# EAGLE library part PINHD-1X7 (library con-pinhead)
PIN HEADER
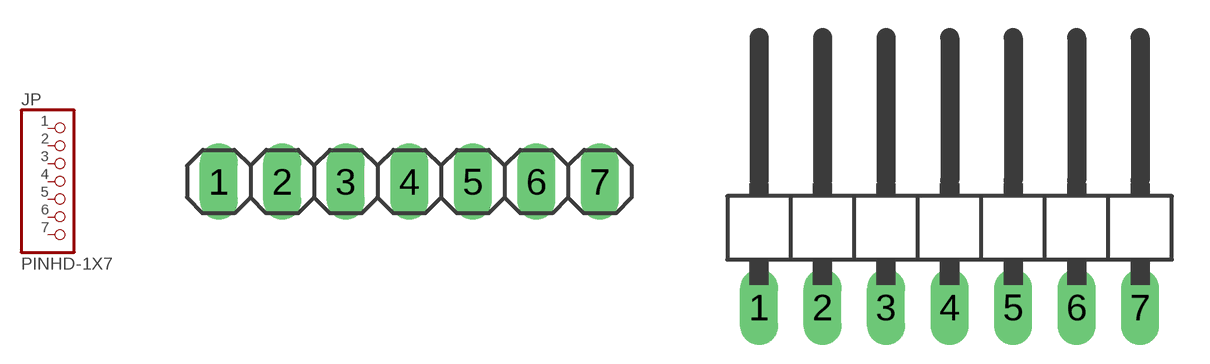
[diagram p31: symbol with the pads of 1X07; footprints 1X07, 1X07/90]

Designator prefix JP

## PINHD-1X7_2.54  [1X07]
1  1  pas
2  2  pas
3  3  pas
4  4  pas
5  5  pas
6  6  pas
7  7  pas

## PINHD-1X7_2.54-90°  [1X07/90]
Pads as for 1X07

## PINHD-1X7_2.00  [1X07M]
Pads as for 1X07

## PINHD-1X7_2.54-SMD  [1X07SMD]
Pads as for 1X07

## PINHD-1X7_2.54-SMD-90°  [1X07SMD/90]
Pads as for 1X07

## Footprint 1X07 (pad centres in mm)
PIN HEADER - 2.54
drill 1.016 long: 1 -7.62,0; 2 -5.08,0; 3 -2.54,0; 4 0,0; 5 2.54,0; 6 5.08,0; 7 7.62,0

## Footprint 1X07/90 (pad centres in mm)
PIN HEADER - 2.54 90°
drill 1.016 long: 1 -7.62,-3.81; 2 -5.08,-3.81; 3 -2.54,-3.81; 4 0,-3.81; 5 2.54,-3.81; 6 5.08,-3.81; 7 7.62,-3.81

## Footprint 1X07M (pad centres in mm)
PIN HEADER - 2
drill 0.914 square: 1 -6,0
drill 0.914: 2 -4,0; 3 -2,0; 4 0,0; 5 2,0; 6 4,0; 7 6,0

## Footprint 1X07SMD (pad centres in mm)
PIN HEADER - 2.54 SMD
smd 1.016 x 3.302: 1 -1.27,1.27; 2 1.27,-1.27; 3 3.81,1.27; 4 6.35,-1.27; 5 8.89,1.27; 6 11.43,-1.27; 7 13.97,1.27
